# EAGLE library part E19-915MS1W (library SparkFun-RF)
Chengdu Ebyte E19-915M30S - 915M LoRa (FSK) TRX Using SX1276 This is a 915 MHz LoRa (or optionally FSK) modulated transciver bassed on the Semtech SX1276. It has a high ouput power of 1W an a pre-installed U.FL connector. Can be used with LoRa WAN with DIO0, DIO1, and DIO2 hooked up to controller interrupt inputs SparkFun Products: SAMD21 Pro RF 1W
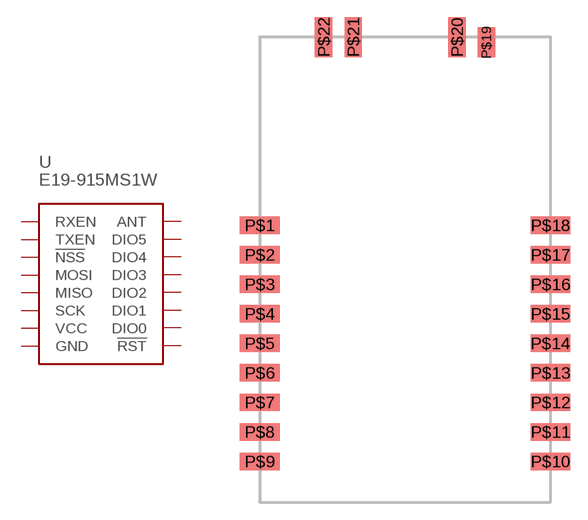
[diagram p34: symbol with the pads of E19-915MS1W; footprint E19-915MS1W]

Designator prefix U

## E19-915MS1W (PROD_ID: IC-14076)  [E19-915MS1W]
P$1  GND
P$2  DIO5
P$3  DIO4
P$4  DIO3
P$5  DIO2
P$6  DIO1
P$7  DIO0
P$8  !RST
P$9  GND
P$10  GND
P$11  VCC
P$12  SCK
P$13  MISO
P$14  MOSI
P$15  !NSS
P$16  TXEN
P$17  RXEN
P$18  GND
P$19  ANT
P$20  GND
P$21  GND
P$22  GND

## Footprint E19-915MS1W (pad centres in mm)
E19-915M30S - 1W 915M TRX Using SX1276 Specifications: Pin count: 22 Pin pitch: Varies Area: 1.15 in x 1.65 in Datasheet referenced for footprint Example device(s): SAMD21 ProRF 1W
smd 3.4 x 1.5: P$1 0,23.82; P$2 0,21.28; P$3 0,18.74; P$4 0,16.2; P$5 0,13.66; P$6 0,11.12; P$7 0,8.58; P$8 0,6.04; P$9 0,3.5; P$10 25,3.5; P$11 25,6.04; P$12 25,8.58; P$13 25,11.12; P$14 24.98,13.66; P$15 25,16.2; P$16 25,18.74; P$17 25,21.28; P$18 25,23.82
smd 1.5 x 2.55: P$19 19.5,39.568
smd 1.5 x 3.4: P$20 16.96,40; P$21 8.04,40; P$22 5.5,40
